(* Logix 5000 DataType export Yaskawa_IN_from_Servo; software revision 17.00 *)

TYPE Yaskawa_IN_from_Servo :   // Structure of data coming from the Yaskawa SigmaLogic controller. v2.4.0
STRUCT
   AlarmText : STRING;   // ServoPack Alarm Code plus Text Description
   b00_Heartbeat : BOOL;
   b01_Alarm : BOOL;   // ServoPack Alarm
   b02_Warning : BOOL;   // ServoPack Warning
   b03_Ready : BOOL;   // ServoPack Ready
   b04_Enabled : BOOL;   // ServoPack Enabled ("Servo On")
   b05_StopComplete : BOOL;
   b06_HomeComplete : BOOL;
   b07_HomeBusy : BOOL;
   b08_HomeActive : BOOL;
   b09_HomeAborted : BOOL;
   b10_HomeError : BOOL;
   b11_MoveAbsComplete : BOOL;
   b12_MoveAbsBusy : BOOL;
   b13_MoveAbsActive : BOOL;
   b14_MoveAbsAborted : BOOL;
   b15_MoveAbsError : BOOL;
   b16_MoveRelComplete : BOOL;
   b17_MoveRelBusy : BOOL;
   b18_MoveRelActive : BOOL;
   b19_MoveRelAborted : BOOL;
   b20_MoveRelError : BOOL;
   b21_JogAtSpeed : BOOL;
   b22_JogBusy : BOOL;
   b23_JogActive : BOOL;
   b24_JogAborted : BOOL;
   b25_JogError : BOOL;
   b26_GearInSync : BOOL;
   b27_GearBusy : BOOL;
   b28_GearActive : BOOL;
   b29_GearAborted : BOOL;
   b30_GearError : BOOL;
   b32_MoveSuperComplete : BOOL;
   b33_MoveSuperBusy : BOOL;
   b34_MoveSuperActive : BOOL;
   b35_MoveSuperAborted : BOOL;
   b36_MoveSuperError : BOOL;
   b37_PowerCycleRequired : BOOL;
   b38_MoveBlend1Complete : BOOL;
   b39_MoveBlend1Busy : BOOL;
   b40_MoveBlend1Active : BOOL;
   b41_MoveBlend1Abort : BOOL;
   b42_MoveBlend1Error : BOOL;
   b43_MoveBlend2Complete : BOOL;
   b44_MoveBlend2Busy : BOOL;
   b45_MoveBlend2Active : BOOL;
   b46_MoveBlend2Abort : BOOL;
   b47_MoveBlend2Error : BOOL;
   b48_RegComplete : BOOL;
   b49_RegBusy : BOOL;
   b50_RegActive : BOOL;
   b51_RegAborted : BOOL;
   b52_RegError : BOOL;
   b53_ResetAbsEncoderActive : BOOL;
   b54_ResetAbsEncoderBusy : BOOL;
   b55_ResetAbsEncoderDone : BOOL;
   b56_ResetAbsEncoderError : BOOL;
   b57_SeqRunning : BOOL;
   b58_RegSensorNotReached : BOOL;
   b59_SeqEditError : BOOL;
   b60_SeqEditDone : BOOL;
   b61_TorqueAtTorque : BOOL;
   b62_TorqueBusy : BOOL;
   b63_TorqueActive : BOOL;
   b64_TorqueAborted : BOOL;
   b65_TorqueError : BOOL;
   b66_ControllerAlarm : BOOL;
   b67_ApplicationError : BOOL;
   b68_AxisAtStandStill : BOOL;
   b69_TestModeActive : BOOL;
   b70_ServoParamsOK : BOOL;
   b71_SetFwdTorqueLimitDone : BOOL;
   b72_SetRevTorqueLimitDone : BOOL;
   Position : DINT;
   Speed : DINT;
   Torque : DINT;
   HomeErrorID : INT;
   MoveAbsErrorID : INT;
   MoveRelErrorID : INT;
   JogErrorID : INT;
   GearErrorID : INT;
   MoveSuperErrorID : INT;
   ServoAlarmID : INT;
   ServoWarningID : INT;
   ControllerAlarmID : DINT;
   AxisGenAlarmID : DINT;
   MoveBlend1ErrorID : INT;
   MoveBlend2ErrorID : INT;
   ResetAbsEncoderErrorID : INT;
   FunctionBlockErrorID : INT;
   TorqueErrorID : INT;
   RegErrorID : INT;
   SeqCurrentStep : INT;
   FlagStatusBit1 : DINT;   // Flag Status. 1..64 are General Flags, Bits 0..31 correspond to Flag 1..32
   FlagStatusBit2 : DINT;   // Flag Status cont. 1..64 are General Flags, Bits 0..31 correspond to Flag 33..64
   IOStatusBits : DINT;   // Digital IO Status. Bits 0-7, CN13 Inputs 0-7, Used as Flag 65-72. Bits 8-15, CN13 Outputs 0-7, Used as Flag 73-80. Bits 16-22, CN1 Inputs 0-6, Used as Flag 81-87. Bits 23-25, CN1 Outputs 0-4, Used as Flag 88-92.
   HSI_Moving : BOOL;
   HSI_Dwelling : BOOL;
   HSI_Done : BOOL;
   HSI_Busy : BOOL;
   HSI_Error : BOOL;
   HSI_ErrorCode : INT;
   PLS_Running : BOOL;
   PLS_SwitchStatus1 : BOOL;
   PLS_SwitchStatus2 : BOOL;
   PLS_SwitchStatus3 : BOOL;
   PLS_SwitchStatus4 : BOOL;
   PLS_Busy : BOOL;
   PLS_Error : BOOL;
   PLS_ErrorCode : INT;
   SetClock_Done : BOOL;
   SetClock_Busy : BOOL;
   SetClock_Error : BOOL;
   SetClock_ErrorID : INT;
   SoftwareVersion : DINT;
   FirmwareVersion : DINT;
   CommandedPos : DINT;
   CommandedPosNonCyc : DINT;
   CommandedSpeed : DINT;
   Clock_Year : INT;
   Clock_Month : INT;
   Clock_Day : INT;
   Clock_Hour : INT;
   Clock_Minute : INT;
   Clock_Second : INT;
   AnalogInput : REAL;   // CN13, AI_01 [v]
   BrakeBypassActive : BOOL;
   ForwardTorqueLimit : DINT;
   ReverseTorqueLimit : DINT;
END_STRUCT
END_TYPE
